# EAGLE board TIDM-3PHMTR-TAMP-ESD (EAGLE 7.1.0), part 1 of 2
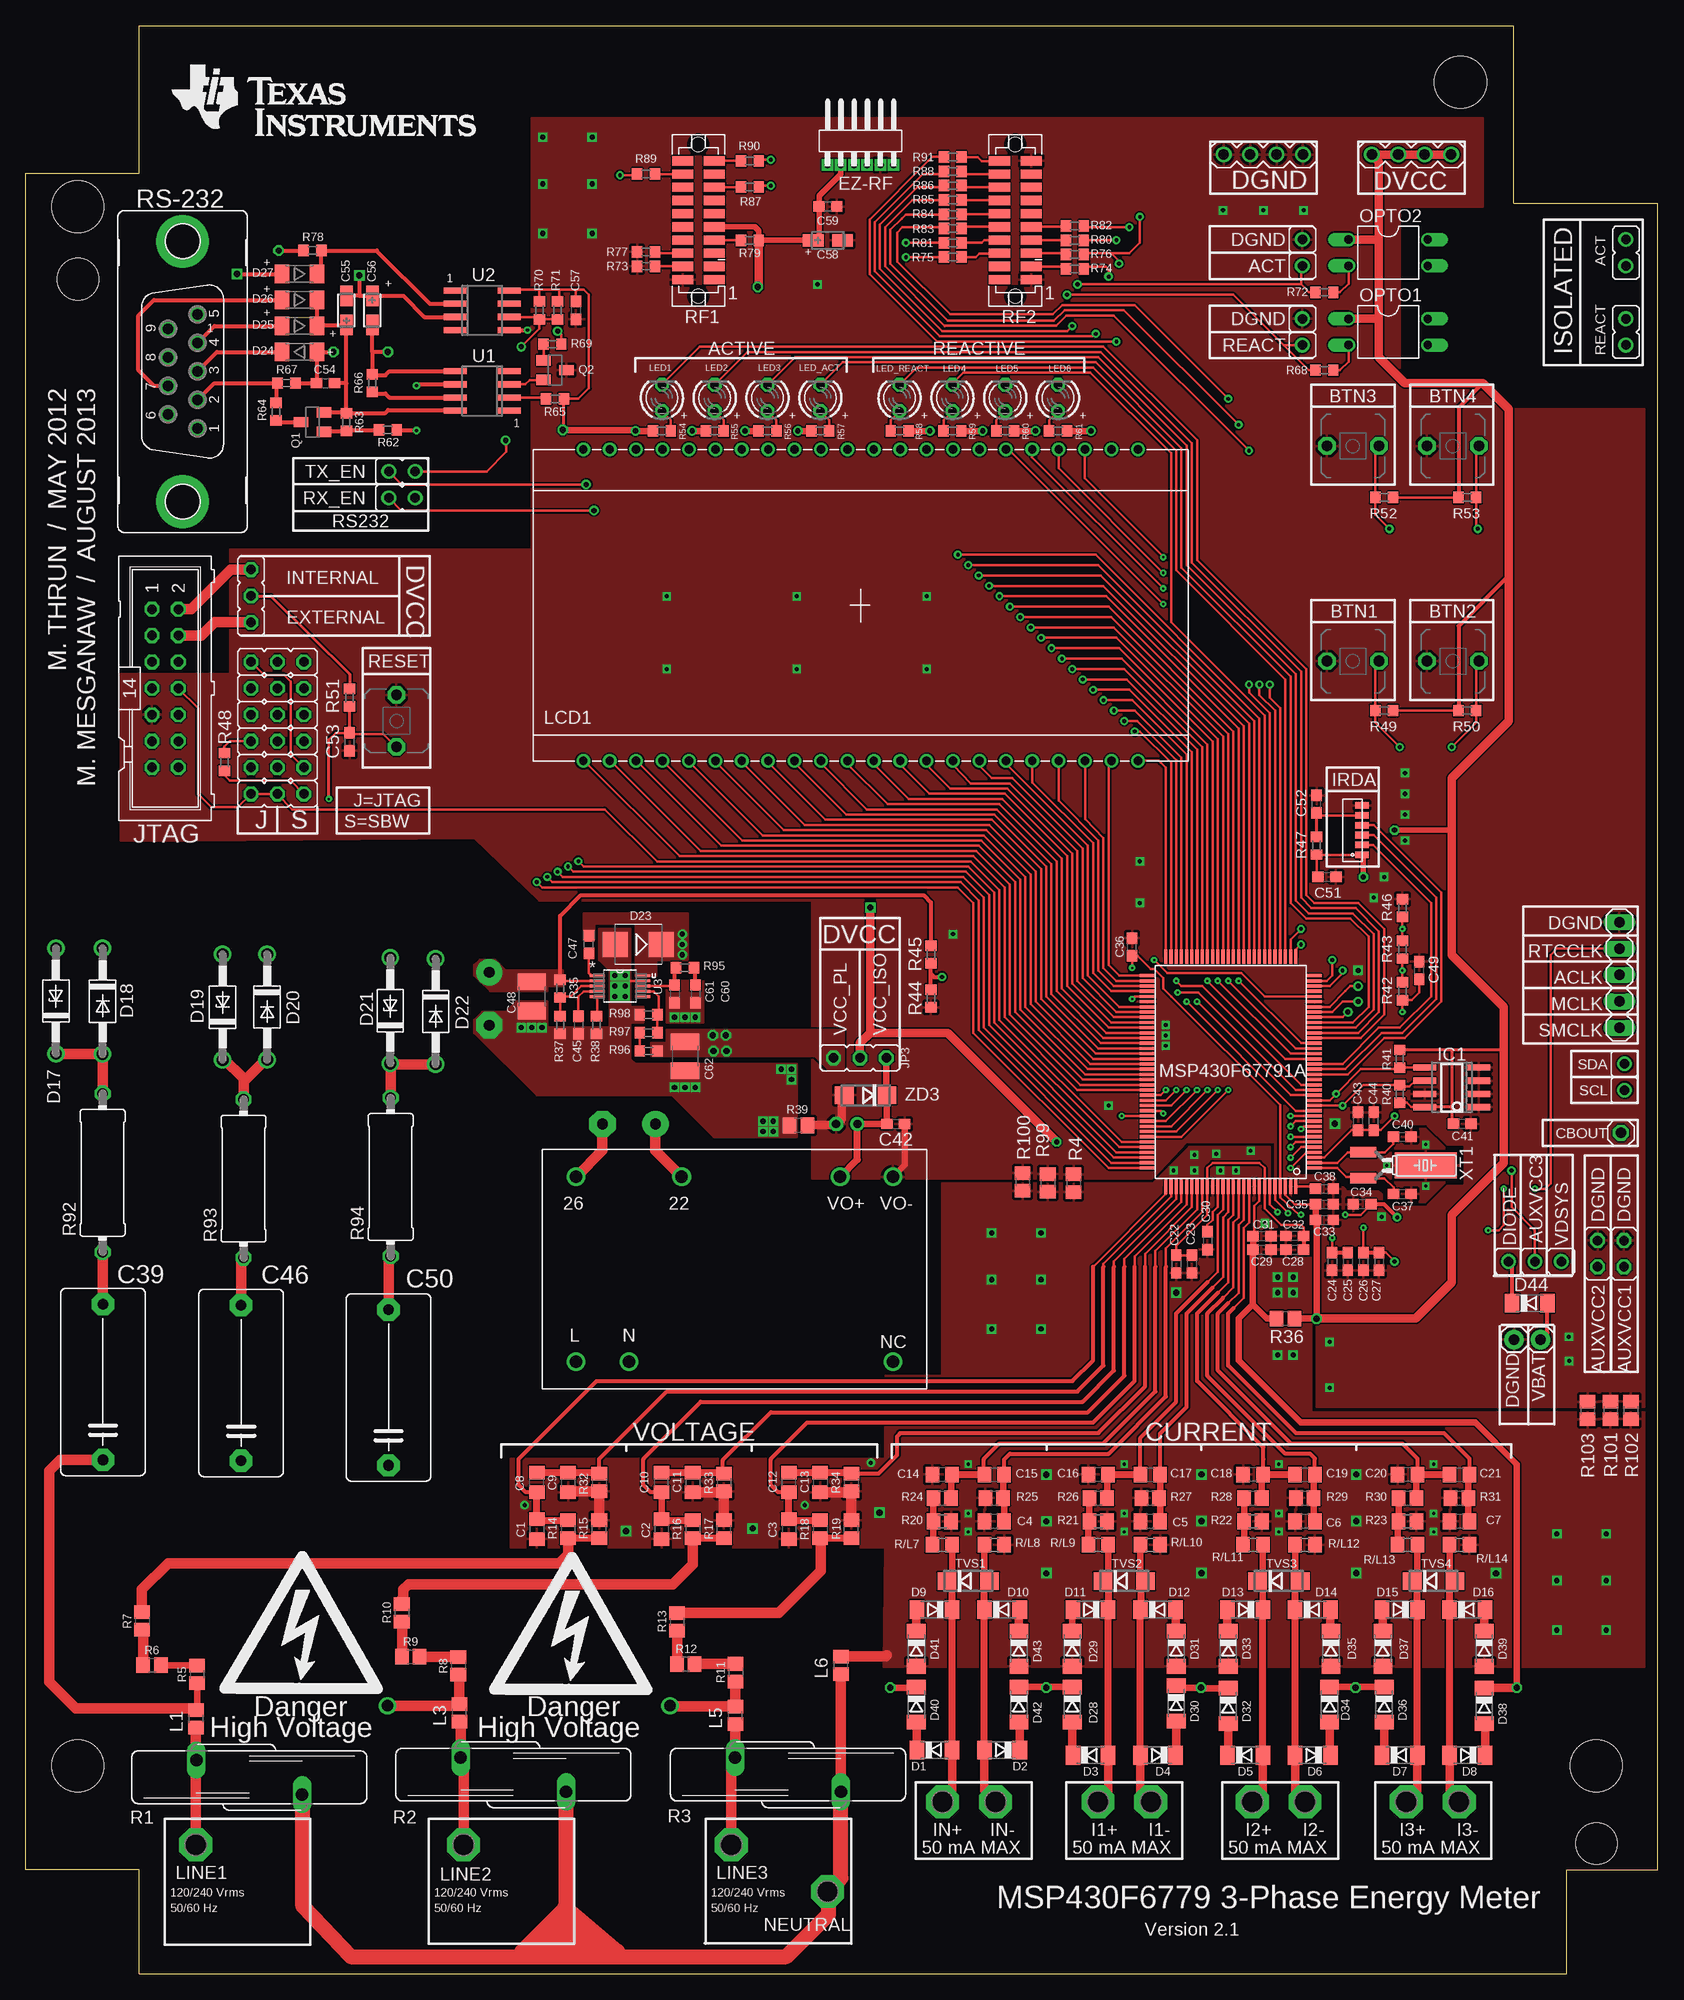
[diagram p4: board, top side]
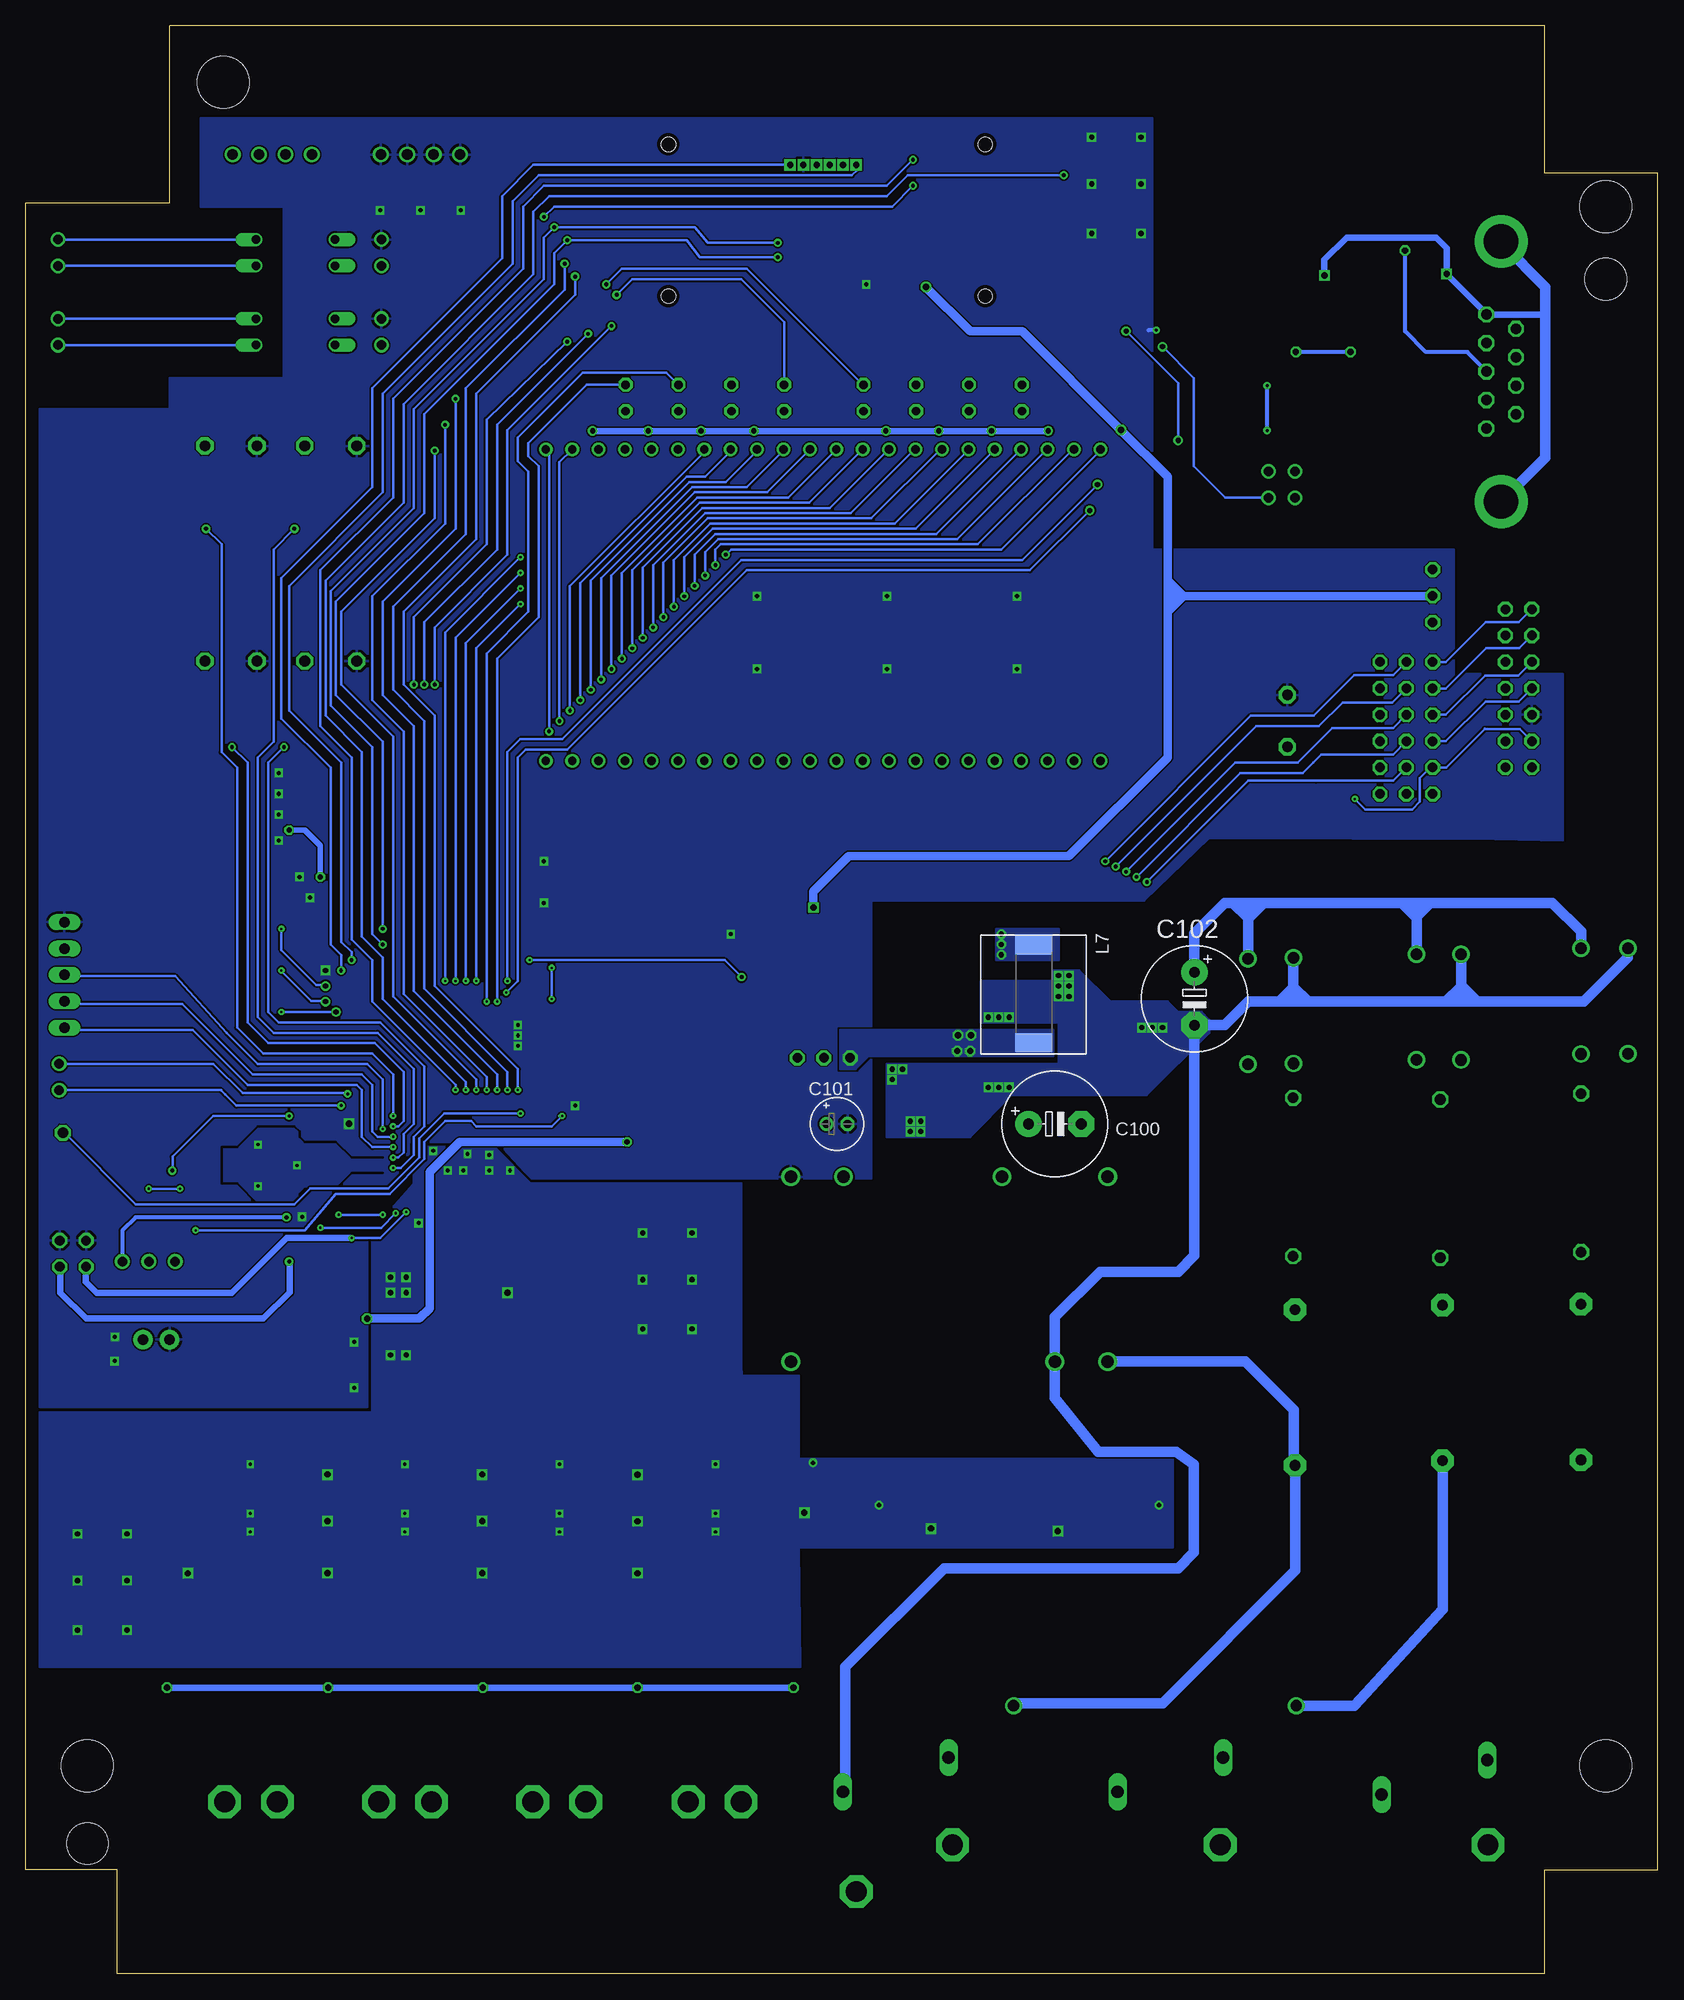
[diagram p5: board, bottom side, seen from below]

Size 156.94 x 187.36 mm. Coordinates in mm from the lower left corner, seen from the top.
Outline: 148.18,0 148.18,10 156.94,10 156.94,170.29 143.1,170.29 143.1,187.36 10.88,187.36 10.88,173.2 0,173.2 0,10 10.88,10 10.88,0 148.18,0
Copper layers (1*16): Top 0.0356mm / dielectric 1.5011mm / Bottom 0.0356mm
Design rules "typical_4pcb *": minimum track width 10mil, minimum drill 15mil, track to track 6mil, track to pad 6mil, pad to pad 6mil, via to via 6mil, smd to smd 6mil, copper to edge 15mil, drill to drill 8mil, minimum pad ring 10mil, minimum via ring 8mil, stop-mask expansion 4mil, vias tented up to drill 25mil, thermal gap 10mil
Holes 5 mm at 137.97,181.95 5,169.99 5,20 151.04,20
Holes 4 mm at 5,163 151.04,12.5
tRestrict: 20 lines
bRestrict: 19 lines

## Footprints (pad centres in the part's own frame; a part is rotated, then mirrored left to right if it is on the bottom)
JP1 = drill 0.914: 1 0,-1.27; 2 0,1.27
JP2 = drill 0.914: 1 -2.54,0; 2 0,0; 3 2.54,0
PBTH = drill 1.016 pad 1.676 octagon: 1 -0.001,0.001; 2 5.001,0.001
C0805 = smd 1.3 x 1.5: 1 -0.95,0; 2 0.95,0
C0603 = smd 1.1 x 1: 1 -0.85,0; 2 0.85,0
C15B8 = drill 1.016 pad 2.159 octagon: 1 -7.493,0; 2 7.493,0
C1210 = smd 1.6 x 2.7: 1 -1.4,0; 2 1.4,0
CT3216 = smd 2 x 1.2: + 1.4,0; - -1.4,0
CT3216' = smd 2 x 1.2: + -1.4,0; - 1.4,0
E5-10,5 = drill 1.016 pad 2.54: + -2.54,0 | drill 1.016 pad 2.54 octagon: - 2.54,0
E2-5 = drill 0.813 pad 1.27: + -1.016,0 | drill 0.813 pad 1.27 octagon: - 1.016,0
SOD80C = smd 1.4 x 1.8: A 1.7,0; C -1.7,0
DO41Z10 = drill 1.118: A 5.08,0; C -5.08,0
DO41-10 = drill 1.118: A 5.08,0; C -5.08,0
SMB = smd 2.4 x 2.4: A 2.2,0; C -2.2,0
SOD80 = smd 1.4 x 1.8: 1 -1.7,0; 2 1.7,0
MA04-1 = drill 1.016: 1 -3.81,0; 2 -1.27,0; 3 1.27,0; 4 3.81,0
SL127L6_MPE = drill 0.6 pad 0.889 square: 1 -3.17,0.07; 2 -1.91,0.07; 3 -0.63,0.07; 4 0.63,0.07; 5 1.91,0.07; 6 3.18,0.07
1X02 = drill 1.016 pad 1.88: 1 0,0; 2 2.54,0
P1-20 = drill 2.007 pad 3.15 octagon: TP 0,0
SO-08 = smd 0.6 x 2.2: 1 -1.905,-2.6; 2 -0.635,-2.6; 3 0.635,-2.6; 4 1.905,-2.6; 5 1.905,2.6; 6 0.635,2.6; 7 -0.635,2.6; 8 -1.905,2.6
TFBS4711 = smd 0.64 x 1.27: P$1 0.625,0.635; P$2 1.575,0.635; P$3 2.525,0.635; P$4 3.475,0.635; P$5 4.425,0.635; P$6 5.375,0.635
JP2' = drill 0.914 octagon: 1 -2.54,0; 2 0,0; 3 2.54,0
1X01 = drill 1.016 octagon: 1 0,0
ML14 = drill 0.914 octagon: 1 -7.62,-1.27; 2 -7.62,1.27; 3 -5.08,-1.27; 4 -5.08,1.27; 5 -2.54,-1.27; 6 -2.54,1.27; 7 0,-1.27; 8 0,1.27; 9 2.54,-1.27; 10 2.54,1.27; 11 5.08,-1.27; 12 5.08,1.27; 13 7.62,-1.27; 14 7.62,1.27
R0805 = smd 1.3 x 1.5: 1 -0.85,0; 2 0.85,0
INDUCTOR_POWER_SUPPLY_6779 = smd 3.556 x 1.778: 1 -3.81,-4.64; 2 -3.81,4.758
TI_160SEG_LCD = drill 0.8: 1 4.826,0; 2 7.366,0; 3 9.906,0; 4 12.446,0; 5 14.986,0; 6 17.526,0; 7 20.066,0; 8 22.606,0; 9 25.146,0; 10 27.686,0; 11 30.226,0; 12 32.766,0; 13 35.306,0; 14 37.846,0; 15 40.386,0; 16 42.926,0; 17 45.466,0; 18 48.006,0; 19 50.546,0; 20 53.086,0; 21 55.626,0; 22 58.166,0; 23 58.166,29.972; 24 55.626,29.972; 29 42.926,29.972; 30 40.386,29.972; 31 37.846,29.972; 32 35.306,29.972; 33 32.766,29.972; 34 30.226,29.972; 35 27.686,29.972; 36 25.146,29.972; 37 22.606,29.972; 38 20.066,29.972; 39 17.526,29.972; 40 14.986,29.972; 41 12.446,29.972; 42 9.906,29.972; 43 7.366,29.972; 44 4.826,29.972; COM0 45.466,29.972; COM1 48.006,29.972; COM2 50.546,29.972; COM3 53.086,29.972
LED3MM = drill 0.813 octagon: A -1.27,0; K 1.27,0
PEU128 = smd 0.3 x 1.4: 1 -9,-7.8; 2 -8.5,-7.8; 3 -8,-7.8; 4 -7.5,-7.8; 5 -7,-7.8; 6 -6.5,-7.8; 7 -6,-7.8; 8 -5.5,-7.8; 9 -5,-7.8; 10 -4.5,-7.8; 11 -4,-7.8; 12 -3.5,-7.8; 13 -3,-7.8; 14 -2.5,-7.8; 15 -2,-7.8; 16 -1.5,-7.8; 17 -1,-7.8; 18 -0.5,-7.8; 19 0,-7.8; 20 0.5,-7.8; 21 1,-7.8; 22 1.5,-7.8; 23 2,-7.8; 24 2.5,-7.8; 25 3,-7.8; 26 3.5,-7.8; 27 4,-7.8; 28 4.5,-7.8; 29 5,-7.8; 30 5.5,-7.8; 31 6,-7.8; 32 6.5,-7.8; 33 7,-7.8; 34 7.5,-7.8; 35 8,-7.8; 36 8.5,-7.8; 37 9,-7.8; 38 9.5,-7.8; 65 9.5,8.3; 66 9,8.3; 67 8.5,8.3; 68 8,8.3; 69 7.5,8.3; 70 7,8.3; 71 6.5,8.3; 72 6,8.3; 73 5.5,8.3; 74 5,8.3; 75 4.5,8.3; 76 4,8.3; 77 3.5,8.3; 78 3,8.3; 79 2.5,8.3; 80 2,8.3; 81 1.5,8.3; 82 1,8.3; 83 0.5,8.3; 84 0,8.3; 85 -0.5,8.3; 86 -1,8.3; 87 -1.5,8.3; 88 -2,8.3; 89 -2.5,8.3; 90 -3,8.3; 91 -3.5,8.3; 92 -4,8.3; 93 -4.5,8.3; 94 -5,8.3; 95 -5.5,8.3; 96 -6,8.3; 97 -6.5,8.3; 98 -7,8.3; 99 -7.5,8.3; 100 -8,8.3; 101 -8.5,8.3; 102 -9,8.3 | smd 1.4 x 0.3: 39 11.3,-6; 40 11.3,-5.5; 41 11.3,-5; 42 11.3,-4.5; 43 11.3,-4; 44 11.3,-3.5; 45 11.3,-3; 46 11.3,-2.5; 47 11.3,-2; 48 11.3,-1.5; 49 11.3,-1; 50 11.3,-0.5; 51 11.3,0; 52 11.3,0.5; 53 11.3,1; 54 11.3,1.5; 55 11.3,2; 56 11.3,2.5; 57 11.3,3; 58 11.3,3.5; 59 11.3,4; 60 11.3,4.5; 61 11.3,5; 62 11.3,5.5; 63 11.3,6; 64 11.3,6.5; 103 -10.8,6.5; 104 -10.8,6; 105 -10.8,5.5; 106 -10.8,5; 107 -10.8,4.5; 108 -10.8,4; 109 -10.8,3.5; 110 -10.8,3; 111 -10.8,2.5; 112 -10.8,2; 113 -10.8,1.5; 114 -10.8,1; 115 -10.8,0.5; 116 -10.8,0; 117 -10.8,-0.5; 118 -10.8,-1; 119 -10.8,-1.5; 120 -10.8,-2; 121 -10.8,-2.5; 122 -10.8,-3; 123 -10.8,-3.5; 124 -10.8,-4; 125 -10.8,-4.5; 126 -10.8,-5; 127 -10.8,-5.5; 128 -10.8,-6
DIL04 = drill 0.813 offset: 1 -1.27,-3.81; 2 1.27,-3.81; 3 1.27,3.81; 4 -1.27,3.81
SOT23-BEC = smd 1 x 1.4: B -0.95,-1.1; C 0,1.1; E 0.95,-1.1
S20K275 = drill 1.194 long: 1 -1.651,-5.08; 2 1.651,5.08
R0603 = smd 1 x 1.1: 1 -0.85,0; 2 0.85,0
0414/15 = drill 1.016 octagon: 1 -7.62,0; 2 7.62,0
R0805' = smd 1.3 x 1.5: 1 -0.95,0; 2 0.95,0
TFM-110-02-SM-D-A-K = smd 2.032 x 0.889: 1 -1.524,5.715; 2 1.524,5.715; 3 -1.524,4.445; 4 1.524,4.445; 5 -1.524,3.175; 6 1.524,3.175; 7 -1.524,1.905; 8 1.524,1.905; 9 -1.524,0.635; 10 1.524,0.635; 11 -1.524,-0.635; 12 1.524,-0.635; 13 -1.524,-1.905; 14 1.524,-1.905; 15 -1.524,-3.175; 16 1.524,-3.175; 17 -1.524,-4.445; 18 1.524,-4.445; 19 -1.524,-5.715; 20 1.524,-5.715 | hole 1.359: 0,7.303; 0,-7.303
F09VP = drill 1.016 octagon: 1 5.486,1.422; 2 2.743,1.422; 3 0,1.422; 4 -2.743,1.422; 5 -5.486,1.422; 6 4.115,-1.422; 7 1.372,-1.422; 8 -1.372,-1.422; 9 -4.115,-1.422 | drill 3.302 pad 5.08: G1 -12.522,0; G2 12.522,0
JP2Q = drill 0.914 octagon: 1 -1.27,-1.27; 2 -1.27,1.27; 3 1.27,-1.27; 4 1.27,1.27
MA05-1 = drill 1.016 long: 1 -5.08,0; 2 -2.54,0; 3 0,0; 4 2.54,0; 5 5.08,0
DO214AC = smd 1.8 x 1.7: A 2.05,0; C -2.05,0
SO08 = smd 0.6 x 2.2: 1 -1.905,-2.6; 2 -0.635,-2.6; 3 0.635,-2.6; 4 1.905,-2.6; 5 1.905,2.6; 6 0.635,2.6; 7 -0.635,2.6; 8 -1.905,2.6
DGQ10_1P88X1P57 = smd 1.422 x 0.279: 1 -2.184,0.991; 2 -2.184,0.508; 3 -2.184,0; 4 -2.184,-0.508; 5 -2.184,-0.991; 6 2.184,-0.991; 7 2.184,-0.508; 8 2.184,0; 9 2.184,0.508; 10 2.184,0.991
CUI_XR = drill 1.2: 22 10.16,0; 26 0,0; L 0,-17.78; N 5.08,-17.78; NC 30.48,-17.78; VO+ 25.4,0; VO- 30.48,0
CM200T = smd 1 x 2.5: P1 -1.25,-5; P2 1.25,-5 | smd 2.5 x 6: P3 0,1

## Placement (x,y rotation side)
ACT  [JP1]  153.87,165.55 0 top
AUXVCC3  [JP2]  145.13,68.5 0 top
BTN1  [PBTH]  125.13,126.26 0 top
BTN2  [PBTH]  134.74,126.26 0 top
BTN3  [PBTH]  125.13,146.96 0 top
BTN4  [PBTH]  134.74,146.96 0 top
C1  47p  [C0805]  49.13,42.75 270 top
C2  47p  [C0805]  61.13,42.75 270 top
C3  47p  [C0805]  73.38,42.75 270 top
C4  47p  [C0805]  93.13,43.5 180 top
C5  47p  [C0805]  108.13,43.5 180 top
C6  47p  [C0805]  123.01,43.5 180 top
C7  47p  [C0805]  137.88,43.5 180 top
C8  15n  [C0805]  49.13,47.25 90 top
C9  47p  [C0805]  52.13,47.25 270 top
C10  15n  [C0805]  61.13,47.25 90 top
C11  47p  [C0805]  64.13,47.25 270 top
C12  15n  [C0805]  73.38,47.25 90 top
C13  47p  [C0805]  76.38,47.25 270 top
C14  47p  [C0805]  88.13,48 180 top
C15  15n  [C0805]  93.13,48 0 top
C16  47p  [C0805]  103.13,48 180 top
C17  15n  [C0805]  108.13,48 0 top
C18  47p  [C0805]  118.01,48 180 top
C19  15n  [C0805]  123.01,48 0 top
C20  47p  [C0805]  132.88,48 180 top
C21  15n  [C0805]  137.88,48 0 top
C22  4.7uF  [C0603]  110.63,68.25 270 top
C23  100nF  [C0603]  112.13,68.25 270 top
C24  4.7uF  [C0603]  125.63,68.5 270 top
C25  100nF  [C0603]  127.13,68.5 270 top
C26  4.7uF  [C0603]  128.63,68.5 270 top
C27  100nF  [C0603]  130.13,68.5 270 top
C28  100nF  [C0603]  122.03,69.62 180 top
C29  4.7uF  [C0603]  118.88,69.65 0 top
C30  100nF  [C0603]  113.63,70.5 270 top
C31  100nF  [C0603]  118.88,70.95 0 top
C32  4.7uF  [C0603]  122.02,70.96 180 top
C33  100nF  [C0603]  124.88,72.5 0 top
C34  4.7uF  [C0603]  128.51,74 180 top
C35  4.7uF  [C0603]  124.88,74 0 top
C36  100nF  [C0603]  106.38,98.75 90 top
C37  12pF  [C0603]  132.38,75 0 top
C38  0.47uF  [C0603]  124.88,75.5 0 top
C39  0.22uF/305VAC  [C15B8]  7.4,56.91 90 top
C40  12pF  [C0603]  132.38,80.5 0 top
C41  0.1uF  [C0603]  138.13,81.75 180 top
C42  0.1uF  [C0603]  83.66,81.73 0 top
C43  100nF  [C0603]  128.13,82 90 top
C44  0.47uF  [C0603]  129.63,82 90 top
C45  0.01uF  [C0603]  53.13,91.25 270 top
C46  0.22uF/305VAC  [C15B8]  20.69,56.81 90 top
C47  0.1uF  [C0603]  54.13,99 90 top
C48  2.2uF  [C1210]  48.63,94 270 top
C49  4.7uF  [C0603]  134.01,96.5 90 top
C50  0.22uF/305VAC  [C15B8]  34.87,56.38 90 top
C51  4.7uF  [C0603]  125.13,105.5 0 top
C52  0.1uF  [C0603]  124.13,112.5 90 top
C53  0.1uF  [C0603]  31.13,118.5 90 top
C54  0.1uF  [C0603]  28.81,153 0 top
C55  10uF  [CT3216]  30.81,160 270 top
C56  10uF  [CT3216]  33.31,160 90 top
C57  0.1uF  [C0603]  52.88,160 270 top
C58  10uF  [CT3216']  77.13,166.75 0 top
C59  0.1uF  [C0603]  77.13,170 180 top
C60  .056uF  [C0603]  64.38,94.25 270 top
C61  100pF  [C0603]  62.38,94.25 270 top
C62  47uF  [C1210]  63.38,88.25 270 top
C100  4.7u/400V  [E5-10,5]  57.99,81.73 0 bottom
C101  150uF  [E2-5]  78.94,81.73 0 bottom
C102  100uF/100V  [E5-10,5]  44.56,93.78 270 bottom
D1  PMLL4148  [SOD80C]  87.38,21.5 0 top
D2  PMLL4148  [SOD80C]  93.88,21.5 180 top
D3  PMLL4148  [SOD80C]  102.38,21 0 top
D4  PMLL4148  [SOD80C]  108.88,21 180 top
D5  PMLL4148  [SOD80C]  117.26,21 0 top
D6  PMLL4148  [SOD80C]  123.76,21 180 top
D7  PMLL4148  [SOD80C]  132.13,21 0 top
D8  PMLL4148  [SOD80C]  138.63,21 180 top
D9  PMLL4148  [SOD80C]  87.38,35 180 top
D10  PMLL4148  [SOD80C]  93.88,35 0 top
D11  PMLL4148  [SOD80C]  102.38,35 180 top
D12  PMLL4148  [SOD80C]  108.88,35 0 top
D13  PMLL4148  [SOD80C]  117.26,35 180 top
D14  PMLL4148  [SOD80C]  123.76,35 0 top
D15  PMLL4148  [SOD80C]  132.13,35 180 top
D16  PMLL4148  [SOD80C]  138.63,35 0 top
D17  1N4757A  [DO41Z10]  2.87,93.57 90 top
D18  1N4007  [DO41-10]  7.37,93.54 270 top
D19  1N4757A  [DO41Z10]  18.92,92.97 90 top
D20  1N4007  [DO41-10]  23.2,92.99 270 top
D21  1N4757A  [DO41Z10]  35.04,92.63 90 top
D22  1N4007  [DO41-10]  39.41,92.54 270 top
D23  B160  [SMB]  58.88,99 180 top
D24  LL103A  [SOD80]  26.31,156 0 top
D25  LL103A  [SOD80]  26.31,158.5 180 top
D26  LL103A  [SOD80]  26.31,161 180 top
D27  LL103A  [SOD80]  26.31,163.5 180 top
D28  PMLL4148  [SOD80C]  100.63,25.88 270 top
D29  PMLL4148  [SOD80C]  100.63,31.25 270 top
D30  PMLL4148  [SOD80C]  110.63,26 270 top
D31  PMLL4148  [SOD80C]  110.63,31.25 270 top
D32  PMLL4148  [SOD80C]  115.63,25.75 270 top
D33  PMLL4148  [SOD80C]  115.63,31.25 270 top
D34  PMLL4148  [SOD80C]  125.38,25.88 270 top
D35  PMLL4148  [SOD80C]  125.51,31.25 270 top
D36  PMLL4148  [SOD80C]  130.63,25.88 270 top
D37  PMLL4148  [SOD80C]  130.51,31.25 270 top
D38  PMLL4148  [SOD80C]  140.26,25.75 270 top
D39  PMLL4148  [SOD80C]  140.26,31.25 270 top
D40  PMLL4148  [SOD80C]  85.63,25.88 270 top
D41  PMLL4148  [SOD80C]  85.63,31.25 270 top
D42  PMLL4148  [SOD80C]  95.51,25.88 270 top
D43  PMLL4148  [SOD80C]  95.51,31.25 270 top
D44  [SOD80C]  144.63,64.5 0 top
DGND  [MA04-1]  119.01,175 0 top
DVCC  [MA04-1]  133.26,175 0 top
EZ-RF  SL127L6TH  [SL127L6_MPE]  80.27,173.93 0 top
HD1  [1X02]  143.13,61 0 top
I1+  TPPAD1-20  [P1-20]  103.11,16.52 90 top
I1-  TPPAD1-20  [P1-20]  108.19,16.52 90 top
I2+  TPPAD1-20  [P1-20]  117.94,16.52 90 top
I2-  TPPAD1-20  [P1-20]  123.02,16.52 90 top
I3+  TPPAD1-20  [P1-20]  132.76,16.52 90 top
I3-  TPPAD1-20  [P1-20]  137.84,16.52 90 top
IC1  24C02CSN  [SO-08]  137.13,85.25 90 top
IN+  TPPAD1-20  [P1-20]  88.16,16.52 90 top
IN-  TPPAD1-20  [P1-20]  93.24,16.52 90 top
IRDA  TFBS4711-TT1  [TFBS4711]  129.13,107 90 top
JP2  [JP1]  153.75,86.25 0 top
JP3  [JP2']  80.21,88.08 180 top
JP4  [JP2']  24.18,113.48 180 top
JP5  [JP2']  24.18,116.02 180 top
JP6  [JP2']  24.18,118.56 180 top
JP7  [JP2']  24.18,121.1 180 top
JP8  [JP2']  24.18,123.64 180 top
JP9  [JP2']  24.18,126.18 180 top
JP10  [JP2']  21.64,132.53 270 top
JP11  [JP1]  122.76,157.93 0 top
JP12  [JP1]  122.76,165.55 0 top
JP13  [1X01]  153.4,80.88 0 top
JTAG  [ML14]  13.39,123.64 270 top
L1  EXCML20A  [R0805]  16.37,24.5 90 top
L3  EXCML20A  [R0805]  41.69,25.09 90 top
L5  EXCML20A  [R0805]  68.23,24.83 90 top
L6  EXCML20A  [R0805]  78.39,29.66 90 top
L7  1mH  [INDUCTOR_POWER_SUPPLY_6779]  63.84,94.3 180 bottom
LCD1  TI_160SEG_LCD  [TI_160SEG_LCD]  48.78,116.66 0 top
LED1  [LED3MM]  61.16,151.58 90 top
LED2  [LED3MM]  66.24,151.58 90 top
LED3  [LED3MM]  71.32,151.58 90 top
LED4  [LED3MM]  89.1,151.58 90 top
LED5  [LED3MM]  94.18,151.58 90 top
LED6  [LED3MM]  99.26,151.58 90 top
LED_ACT  [LED3MM]  76.4,151.58 90 top
LED_REACT  [LED3MM]  84.02,151.58 90 top
LINE1  TPPAD1-20  [P1-20]  16.33,12.38 90 top
LINE2  TPPAD1-20  [P1-20]  42.08,12.38 90 top
LINE3  TPPAD1-20  [P1-20]  67.83,12.38 90 top
MSP430F67791A  MSP430F6779IPEU  [PEU128]  116.13,86.5 90 top
NEUTRAL  TPPAD1-20  [P1-20]  77.08,7.88 90 top
OPTO1  TIL191  [DIL04]  131.01,157.93 270 top
OPTO2  TIL191  [DIL04]  131.01,165.55 270 top
Q1  BC857BSMD  [SOT23-BEC]  27.56,149.25 90 top
Q2  BC857BSMD  [SOT23-BEC]  50.88,154.25 270 top
R1  S20K275  [S20K275]  21.48,18.88 90 top
R2  S20K275  [S20K275]  46.88,19.14 90 top
R3  S20K275  [S20K275]  73.29,19.14 90 top
R4  0  [R0805]  100.76,76.03 270 top
R5  330k  [R0805]  16.44,28.78 270 top
R6  330k  [R0805]  12.12,29.66 0 top
R7  330k  [R0805]  11.17,33.92 270 top
R8  330k  [R0805]  41.57,29.61 270 top
R9  330k  [R0805]  37.02,30.49 0 top
R10  330k  [R0805]  36.14,34.69 270 top
R11  330k  [R0805]  68.26,28.94 270 top
R12  330k  [R0805]  63.47,29.79 0 top
R13  330k  [R0805]  62.62,33.83 270 top
R14  1k  [R0805]  52.13,42.75 270 top
R15  2.37K  [R0805]  55.13,42.75 90 top
R16  1k  [R0805]  64.13,42.75 270 top
R17  2.37K  [R0805]  67.13,42.75 90 top
R18  1k  [R0805]  76.38,42.75 270 top
R19  2.37K  [R0805]  79.38,42.75 90 top
R20  12.4  [R0805]  88.13,43.5 180 top
R21  12.4  [R0805]  103.13,43.5 180 top
R22  12.4  [R0805]  118.01,43.5 180 top
R23  12.4  [R0805]  132.88,43.5 180 top
R24  1k  [R0805]  88.13,45.75 0 top
R25  1k  [R0805]  93.13,45.75 0 top
R26  1k  [R0805]  103.13,45.75 0 top
R27  1k  [R0805]  108.13,45.75 0 top
R28  1k  [R0805]  118.01,45.75 0 top
R29  1k  [R0805]  123.01,45.75 0 top
R30  1k  [R0805]  132.88,45.75 0 top
R31  1k  [R0805]  137.88,45.75 0 top
R32  1k  [R0805]  55.13,47.25 270 top
R33  1k  [R0805]  67.13,47.25 270 top
R34  1k  [R0805]  79.38,47.25 270 top
R35  1M  [R0603]  51.38,94.75 90 top
R36  10R  [R0805]  121.14,63.01 180 top
R37  33.2K  [R0603]  51.38,91.25 90 top
R38  1M  [R0603]  54.88,91.25 90 top
R39  0  [R0805]  74.3,81.59 180 top
R40  10k  [R0603]  132.13,84.62 270 top
R41  10k  [R0603]  132.13,88 90 top
R42  560k  [R0603]  132.38,94.5 270 top
R43  560k  [R0603]  132.38,98.5 270 top
R44  DNP  [R0603]  87.03,93.79 90 top
R45  DNP  [R0603]  87.03,98.04 90 top
R46  560k  [R0603]  132.38,102.5 270 top
R47  47  [R0603]  124.13,108.5 90 top
R48  330  [R0603]  19.07,116.56 270 top
R49  100K  [R0603]  130.63,121.5 180 top
R50  100K  [R0603]  138.63,121.5 0 top
R51  47K  [R0603]  31.13,122.75 270 top
R52  100K  [R0603]  130.63,142 180 top
R53  100K  [R0603]  138.63,142 0 top
R54  100  [R0603]  61.16,148.41 0 top
R55  100  [R0603]  66.24,148.41 0 top
R56  100  [R0603]  71.32,148.41 0 top
R57  100  [R0603]  76.4,148.41 0 top
R58  100  [R0603]  84.02,148.41 180 top
R59  100  [R0603]  89.1,148.41 180 top
R60  100  [R0603]  94.18,148.41 180 top
R61  100  [R0603]  99.26,148.41 180 top
R62  1k  [R0603]  34.81,148.5 180 top
R63  10k  [R0603]  30.81,149.25 90 top
R64  220  [R0603]  24.06,150.25 270 top
R65  68  [R0603]  50.88,151.5 180 top
R66  DNP  [R0603]  33.31,153 90 top
R67  1.5k  [R0603]  25.06,153 180 top
R68  1k  [R0603]  124.88,154.25 0 top
R69  2.2k  [R0603]  50.63,156.75 180 top
R70  DNP  [R0603]  49.38,160 90 top
R71  2.2k  [R0603]  51.13,160 270 top
R72  1k  [R0603]  124.88,161.75 0 top
R73  0  [R0603]  59.63,164.25 180 top
R74  0  [R0603]  100.88,164 180 top
R75  0  [R0603]  89.13,165.12 180 top
R76  0  [R0603]  100.88,165.38 180 top
R77  0  [R0603]  59.63,165.62 180 top
R78  1k  [R0603]  27.56,165.75 180 top
R79  0  [R0603]  69.63,166.75 180 top
R80  0  [R0603]  100.88,166.75 180 top
R81  0  [R0603]  89.13,166.5 180 top
R82  0  [R0603]  100.88,168.12 180 top
R83  0  [R0603]  89.13,167.88 180 top
R84  0  [R0603]  89.13,169.25 180 top
R85  0  [R0603]  89.13,170.62 180 top
R86  0  [R0603]  89.13,172 180 top
R87  0  [R0603]  69.63,171.88 180 top
R88  0  [R0603]  89.13,173.38 180 top
R89  0  [R0603]  59.63,173.12 180 top
R90  0  [R0603]  69.63,174.38 180 top
R91  0  [R0603]  89.13,174.75 180 top
R92  100  [0414/15]  7.37,77.03 90 top
R93  100  [0414/15]  20.92,76.47 90 top
R94  100  [0414/15]  35.07,76.63 90 top
R95  22.1k  [R0603]  63.38,96.75 180 top
R96  51.1  [R0603]  59.88,88.75 0 top
R97  31.6k  [R0603]  59.88,90.5 180 top
R98  10k  [R0603]  59.88,92.25 0 top
R99  0  [R0805]  98.27,76.06 270 top
R100  0  [R0805]  95.86,76.16 270 top
R101  0  [R0805]  152.4,54.19 270 top
R102  0  [R0805]  154.35,54.19 270 top
R103  0  [R0805]  150.19,54.16 270 top
R/L7  0  [R0805']  88.13,41.25 0 top
R/L8  0  [R0805']  93.13,41.25 180 top
R/L9  0  [R0805']  103.13,41.25 0 top
R/L10  0  [R0805']  108.13,41.25 180 top
R/L11  0  [R0805']  118.01,41.25 0 top
R/L12  0  [R0805']  123.01,41.25 180 top
R/L13  0  [R0805']  132.88,41.25 0 top
R/L14  0  [R0805']  137.88,41.25 180 top
REACT  [JP1]  153.87,157.93 0 top
RESET  [PBTH]  35.63,118 90 top
RF1  [TFM-110-02-SM-D-A-K]  64.67,168.67 180 top
RF2  [TFM-110-02-SM-D-A-K]  95.15,168.67 180 top
RS-232  [F09VP]  15.06,154.12 270 top
RX_EN  [JP1]  36.17,141.97 90 top
SV1  [JP2Q]  152.43,69.25 0 top
SV2  [MA05-1]  153.25,96.06 270 top
TVS1  SMAJ5.0CA  [DO214AC]  90.63,37.75 0 top
TVS2  SMAJ5.0CA  [DO214AC]  105.63,37.75 0 top
TVS3  SMAJ5.0CA  [DO214AC]  120.51,37.75 0 top
TVS4  SMAJ5.0CA  [DO214AC]  135.38,37.75 0 top
TX_EN  [JP1]  36.17,144.51 90 top
U1  PS8802  [SO08]  43.88,152.25 90 top
U2  PS8802  [SO08]  43.88,160 270 top
U3  TPS54060_DGQ_10  [DGQ10_1P88X1P57]  57.13,95 0 top
U$1  CUI_XR  [CUI_XR]  52.91,76.65 0 top
XT1  [CM200T]  133.63,77.75 270 top
ZD3  SMAJ5.0ABCT  [DO214AC]  80.76,84.5 180 top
